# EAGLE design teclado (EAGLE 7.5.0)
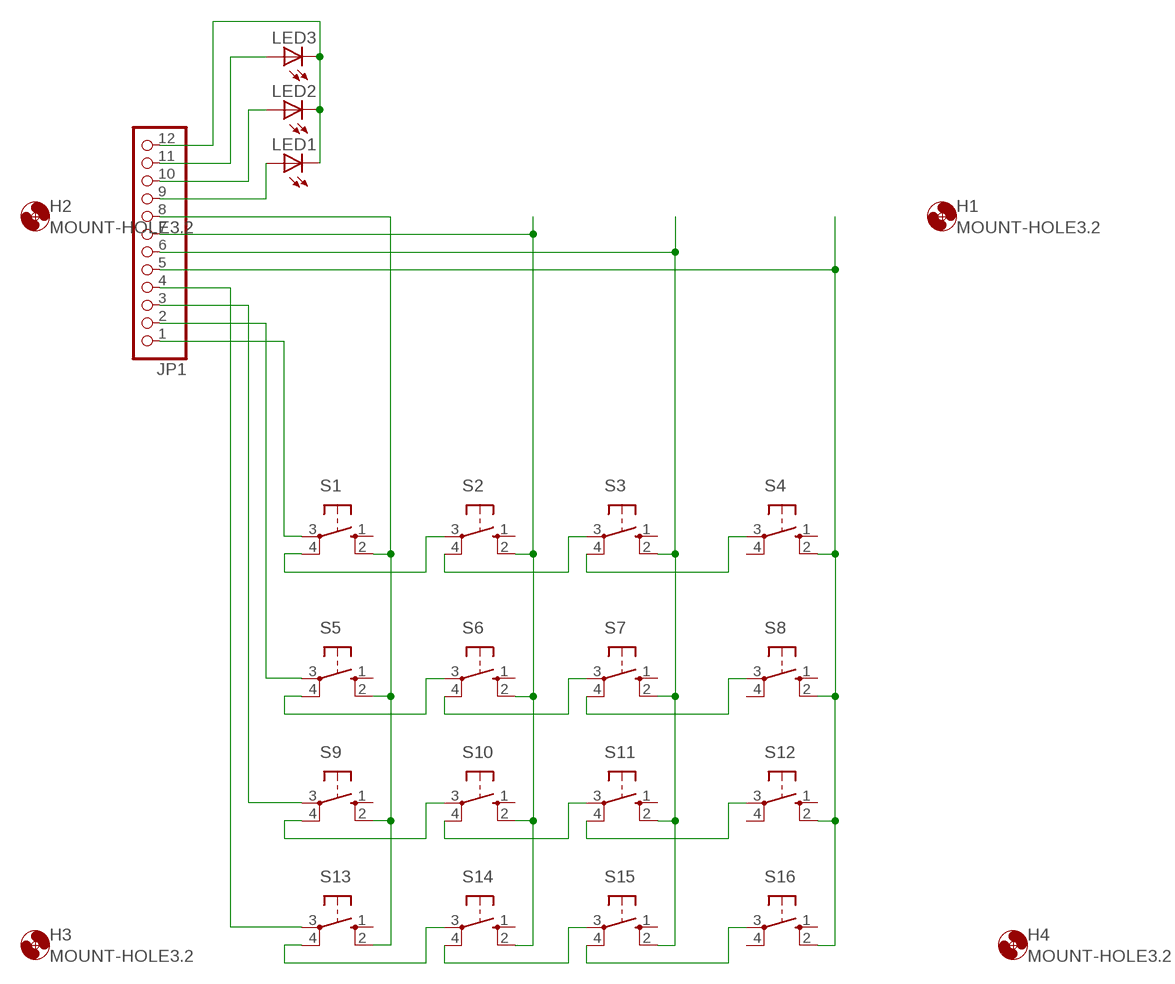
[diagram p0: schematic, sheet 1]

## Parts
H1  MOUNT-HOLE3.2  [3,2]
H2  MOUNT-HOLE3.2  [3,2]
H3  MOUNT-HOLE3.2  [3,2]
H4  MOUNT-HOLE3.2  [3,2]
JP1  PINHD-1X12  [1X12]
LED1  LED5MM  [LED5MM]
LED2  LED5MM  [LED5MM]
LED3  LED5MM  [LED5MM]
S1  10-XX  [B3F-10XX]
S2  10-XX  [B3F-10XX]
S3  10-XX  [B3F-10XX]
S4  10-XX  [B3F-10XX]
S5  10-XX  [B3F-10XX]
S6  10-XX  [B3F-10XX]
S7  10-XX  [B3F-10XX]
S8  10-XX  [B3F-10XX]
S9  10-XX  [B3F-10XX]
S10  10-XX  [B3F-10XX]
S11  10-XX  [B3F-10XX]
S12  10-XX  [B3F-10XX]
S13  10-XX  [B3F-10XX]
S14  10-XX  [B3F-10XX]
S15  10-XX  [B3F-10XX]
S16  10-XX  [B3F-10XX]

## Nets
N$1: JP1.1 S1.3(P)
N$2: JP1.8 S1.2(S1) S5.2(S1) S9.2(S1) S13.2(S1)
N$3: JP1.7 S2.2(S1) S6.2(S1) S10.2(S1) S14.2(S1)
N$4: JP1.6 S3.2(S1) S7.2(S1) S11.2(S1) S15.2(S1)
N$5: JP1.5 S4.2(S1) S8.2(S1) S12.2(S1) S16.2(S1)
N$6: S1.4(P1) S2.3(P)
N$7: S5.4(P1) S6.3(P)
N$8: S9.4(P1) S10.3(P)
N$9: S13.4(P1) S14.3(P)
N$10: S2.4(P1) S3.3(P)
N$11: S6.4(P1) S7.3(P)
N$12: S10.4(P1) S11.3(P)
N$13: S14.4(P1) S15.3(P)
N$14: S3.4(P1) S4.3(P)
N$15: S7.4(P1) S8.3(P)
N$16: S11.4(P1) S12.3(P)
N$17: S15.4(P1) S16.3(P)
N$18: JP1.2 S5.3(P)
N$19: JP1.3 S9.3(P)
N$20: JP1.4 S13.3(P)
N$21: JP1.9 LED1.A
N$22: JP1.10 LED2.A
N$23: JP1.11 LED3.A
N$24: JP1.12 LED1.K(C) LED2.K(C) LED3.K(C)
Unconnected: S1.1(S) S2.1(S) S3.1(S) S4.1(S) S4.4(P1) S5.1(S) S6.1(S) S7.1(S) S8.1(S) S8.4(P1) S9.1(S) S10.1(S) S11.1(S) S12.1(S) S12.4(P1) S13.1(S) S14.1(S) S15.1(S) S16.1(S) S16.4(P1)

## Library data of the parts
H1-H4 = holes:MOUNT-HOLE: MOUNTING HOLE with drill center marker
JP1 = pinhead:PINHD-1X12: PIN HEADER
LED1-LED3 = led:LED: LED
S1-S16 = switch-omron:10-XX: OMRON SWITCH; MPN: B3F-1000; OC_FARNELL: 176432; OC_NEWARK: 36M3542

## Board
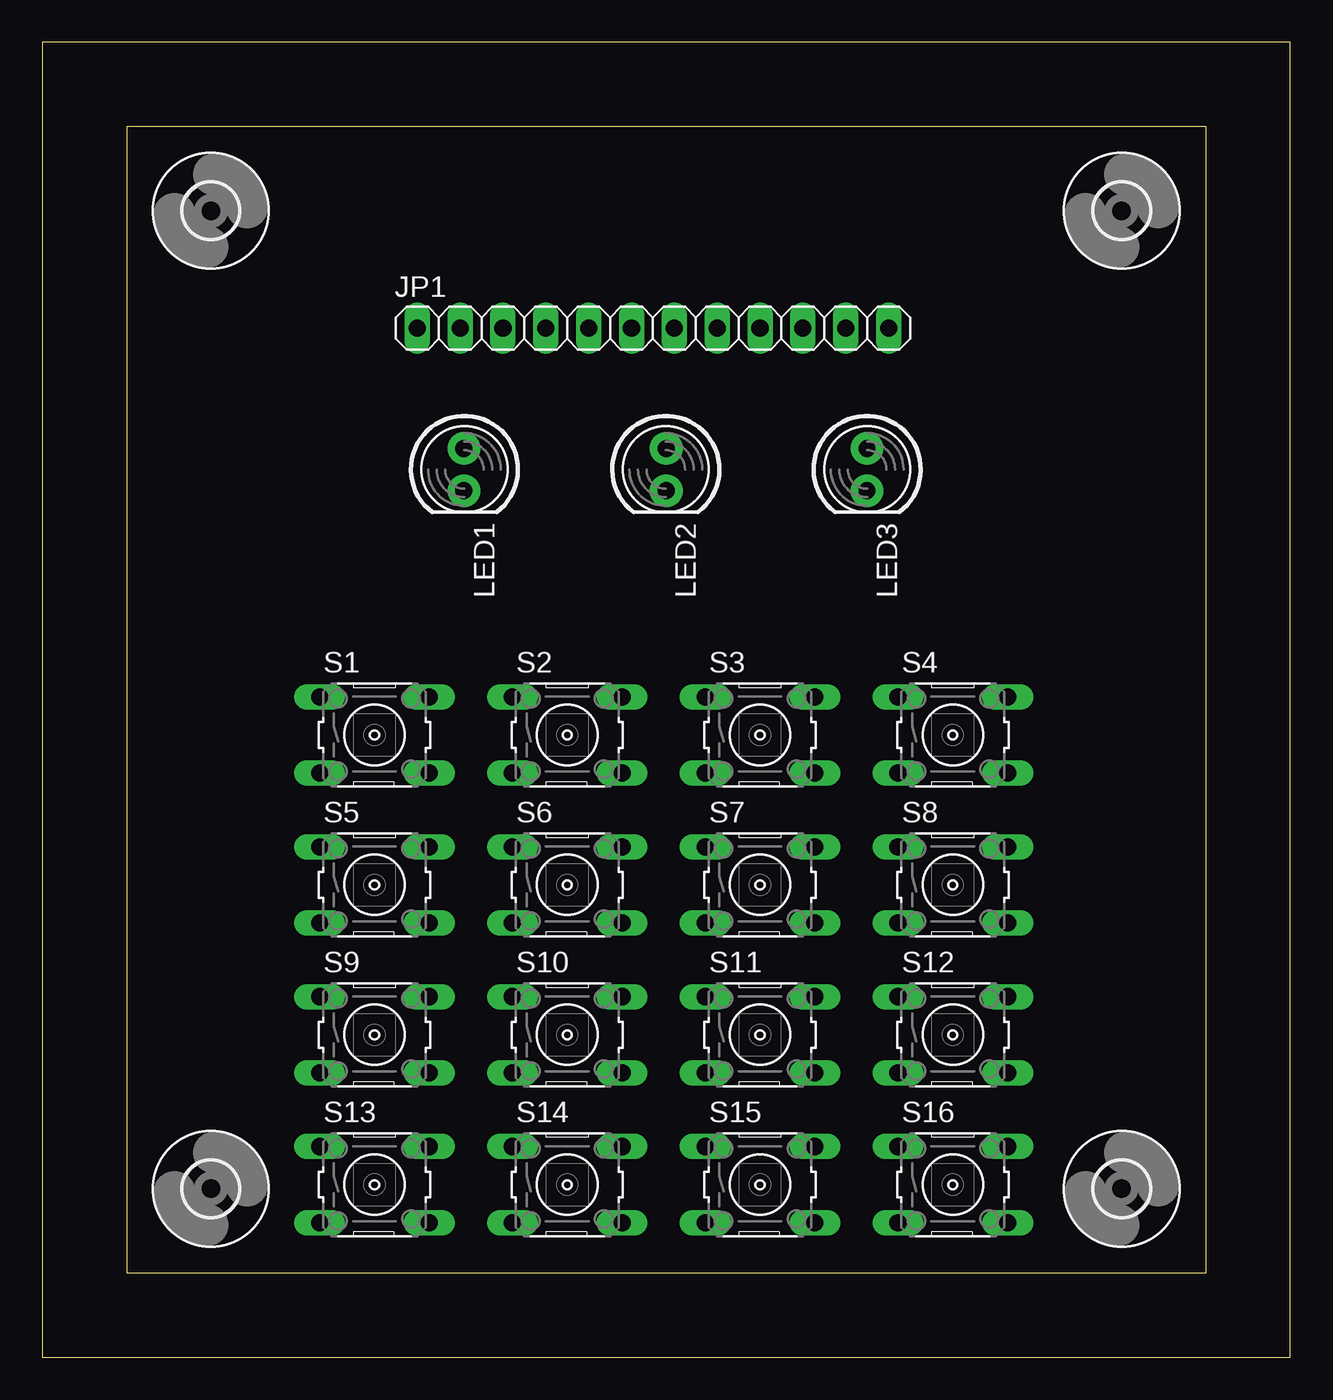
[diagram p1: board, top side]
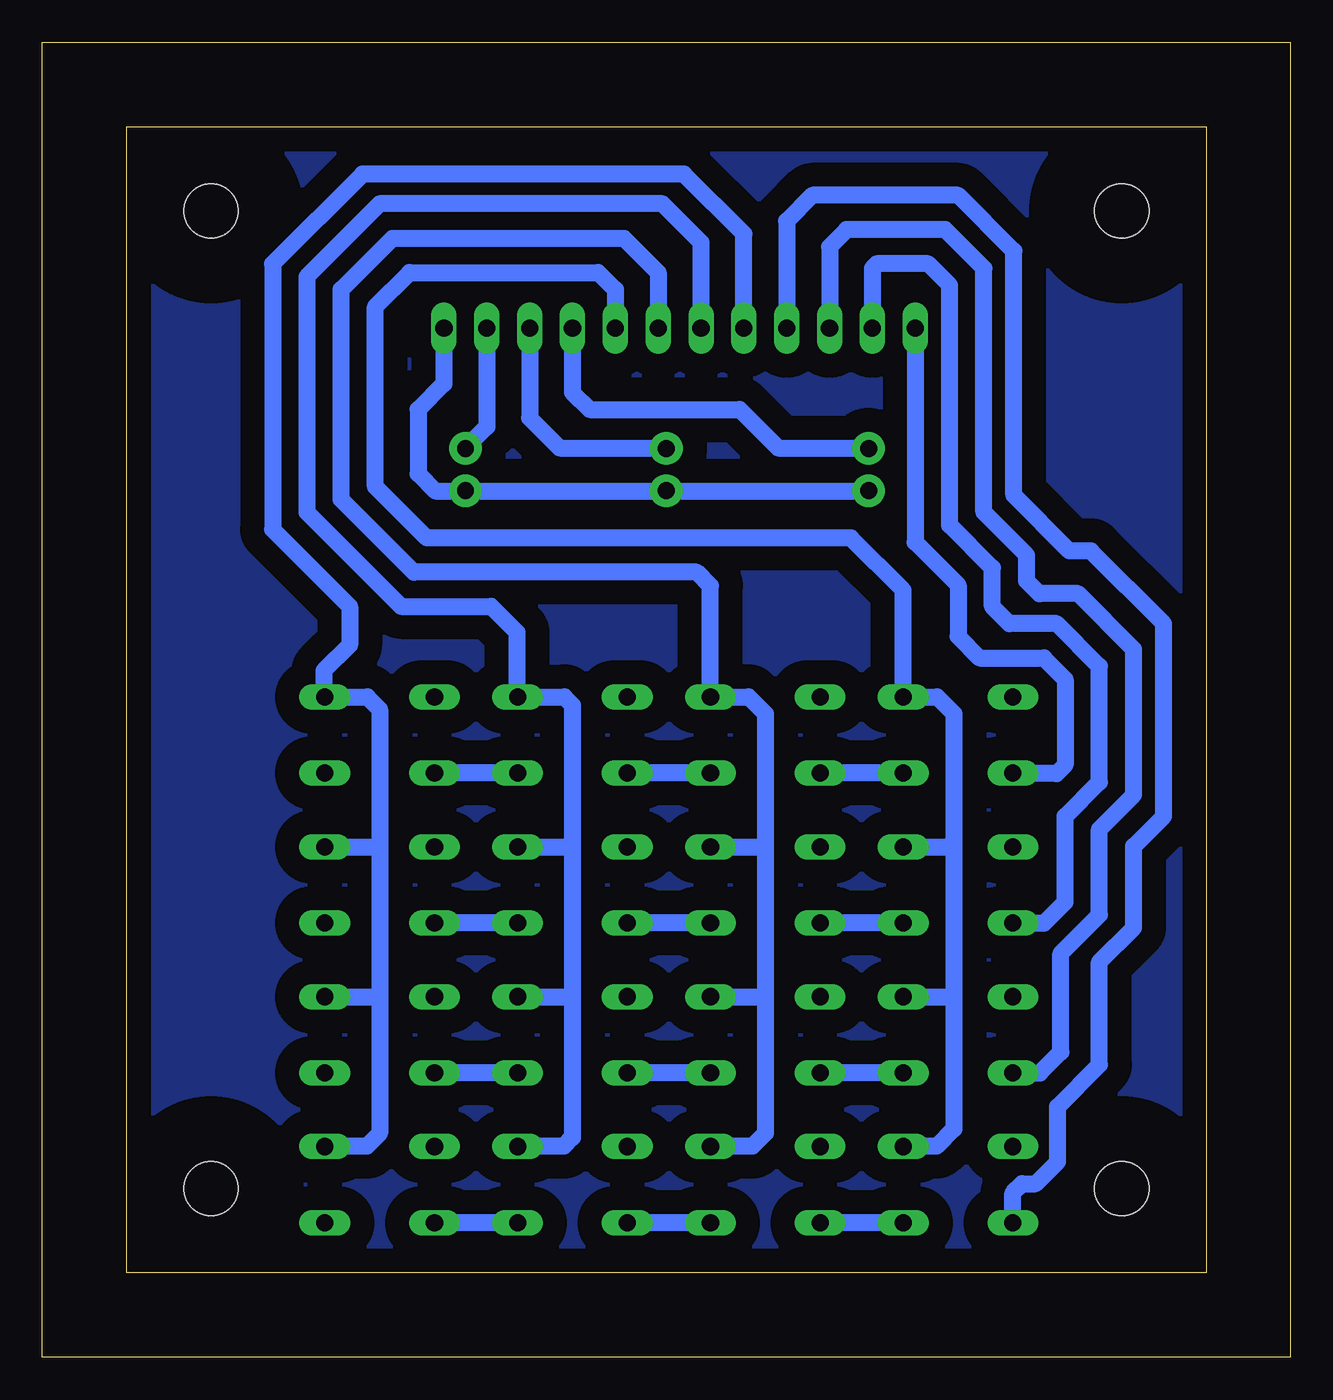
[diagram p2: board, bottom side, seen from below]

Size 74 x 78 mm. Coordinates in mm from the lower left corner, seen from the top.
Outline: 5,5 69,5 69,73 5,73 5,5
Outline: 0,0 74,0 74,78 0,78 0,0
Copper layers (1*16): Top 0.035mm / dielectric 1.5mm / Bottom 0.035mm
Design rules "default": minimum track width 10mil, minimum drill 24mil, track to track 8mil, track to pad 8mil, pad to pad 8mil, via to via 8mil, smd to smd 8mil, copper to edge 40mil, drill to drill 8mil, minimum pad ring 10mil, minimum via ring 8mil, stop-mask expansion 4mil, vias tented up to drill 0mil, thermal gap 10mil

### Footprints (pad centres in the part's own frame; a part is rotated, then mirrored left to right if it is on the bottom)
3,2 = hole 3.2: 0,0
1X12 = drill 1.016 long: 1 -13.97,0; 2 -11.43,0; 3 -8.89,0; 4 -6.35,0; 5 -3.81,0; 6 -1.27,0; 7 1.27,0; 8 3.81,0; 9 6.35,0; 10 8.89,0; 11 11.43,0; 12 13.97,0
LED5MM = drill 0.813 octagon: A -1.27,0; K 1.27,0
B3F-10XX = drill 1.016 long: 1 -3.251,2.261; 2 3.251,2.261; 3 -3.251,-2.261; 4 3.251,-2.261

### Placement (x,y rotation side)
H1  10,68 0 top
H2  64,68 0 top
H3  64,10 0 top
H4  10,10 0 top
JP1  36.21,61.04 0 top
LED1  25.03,52.66 270 top
LED2  36.97,52.66 270 top
LED3  48.91,52.66 270 top
S1  19.7,36.91 0 top
S2  31.13,36.91 0 top
S3  42.56,36.91 0 top
S4  53.99,36.91 0 top
S5  19.7,28.02 0 top
S6  31.13,28.02 0 top
S7  42.56,28.02 0 top
S8  53.99,28.02 0 top
S9  19.7,19.13 0 top
S10  31.13,19.13 0 top
S11  42.56,19.13 0 top
S12  53.99,19.13 0 top
S13  19.7,10.24 0 top
S14  31.13,10.24 0 top
S15  42.56,10.24 0 top
S16  53.99,10.24 0 top

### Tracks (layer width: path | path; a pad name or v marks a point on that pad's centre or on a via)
N$1
  Bottom 1.016: JP1.1 22.24,48.34 19.7,45.8 19.7,42.75 18.43,41.48 14.62,41.48 13.35,40.21 13.35,35.13 13.86,34.62 16.42,34.62 S1.3
N$2
  Bottom 1.016: 19.95,30.56 19.95,38.18 20.95,39.17 S1.2 22.95,45.49 26.05,48.59 51.2,48.59 54.24,51.64 54.24,62.31 52.21,64.34 41.04,64.34 40.02,63.33 JP1.8 | 19.95,30.56 19.95,21.42 | 19.95,21.42 19.95,13.54 20.97,12.53 22.93,12.53 S13.2 | S9.2 19.98,21.39 19.95,21.42 | S5.2 20.23,30.28 19.95,30.56
N$3
  Bottom 1.016: 31.13,30.05 31.13,38.18 32.12,39.17 S2.2 34.38,45.75 35.19,46.56 51.96,46.56 56.28,50.88 56.28,63.33 53.23,66.37 39.51,66.37 37.48,64.34 JP1.7 | 31.13,30.05 31.13,21.42 | 31.13,21.42 31.13,13.29 31.89,12.53 34.36,12.53 S14.2 | S10.2 31.16,21.39 31.13,21.42 | S6.2 31.36,30.28 31.13,30.05
N$4
  Bottom 1.016: 42.56,30.56 42.56,38.69 43.04,39.17 S3.2 45.86,39.22 45.86,43.01 47.39,44.53 52.72,44.53 58.31,50.12 58.31,64.09 53.99,68.41 37.23,68.41 34.94,66.12 JP1.6 | 42.56,30.56 42.56,21.42 | 42.56,21.42 42.56,13.03 43.07,12.53 45.79,12.53 S15.2 | S11.2 42.59,21.39 42.56,21.42 | S7.2 42.84,30.28 42.56,30.56
N$5
  Bottom 1.016: 53.99,30.31 53.99,38.43 54.73,39.17 S4.2 57.29,39.22 57.29,40.72 55.77,42.24 55.77,44.53 60.34,49.1 60.34,64.85 55.01,70.18 35.96,70.18 32.4,66.63 JP1.5 | 53.99,30.31 53.99,21.16 | 53.99,21.16 53.99,13.29 54.75,12.53 57.22,12.53 S16.2 | S12.2 54.22,21.39 53.99,21.16 | S8.2 54.02,30.28 53.99,30.31
N$6
  Bottom 1.016: S1.4 S2.3
N$7
  Bottom 1.016: S5.4 S6.3
N$8
  Bottom 1.016: S9.4 S10.3
N$9
  Bottom 1.016: S13.4 S14.3
N$10
  Bottom 1.016: S2.4 S3.3
N$11
  Bottom 1.016: S6.4 S7.3
N$12
  Bottom 1.016: S10.4 S11.3
N$13
  Bottom 1.016: S14.4 S15.3
N$14
  Bottom 1.016: S3.4 S4.3
N$15
  Bottom 1.016: S7.4 S8.3
N$16
  Bottom 1.016: S11.4 S12.3
N$17
  Bottom 1.016: S15.4 S16.3
N$18
  Bottom 1.016: S5.3 14.6,25.76 13.35,27 13.35,32.08 11.32,34.12 11.32,40.97 13.86,43.51 16.65,43.51 17.67,44.53 17.67,46.82 20.21,49.36 20.21,63.58 21.48,64.85 24.53,64.85 24.78,64.6 JP1.2
N$19
  Bottom 1.016: S9.3 14.85,16.87 13.6,18.11 13.6,23.96 11.32,26.24 11.32,31.32 9.29,33.35 9.29,41.99 12.59,45.29 14.87,45.29 15.64,46.05 15.64,47.58 18.18,50.12 18.18,64.6 20.46,66.88 26.3,66.88 27.32,65.87 JP1.3
N$20
  Bottom 1.016: JP1.4 29.86,67.39 28.34,68.91 19.7,68.91 16.4,65.61 16.4,51.13 13.1,47.83 11.83,47.83 7.51,43.51 7.51,32.08 9.29,30.31 9.29,25.48 11.32,23.45 11.32,17.35 13.8,14.87 13.8,11.6 15.1,10.3 15.9,10.3 16.45,9.75 S13.3
N$21
  Bottom 1.016: JP1.9 42.56,57.23 41.54,56.21 32.65,56.21 30.37,53.93 LED1.A
N$22
  Bottom 1.016: JP1.10 45.1,55.71 43.32,53.93 LED2.A
N$23
  Bottom 1.016: JP1.11 47.64,55.2 LED3.A
N$24
  Bottom 1.016: JP1.12 50.18,57.74 51.7,56.21 51.7,52.4 50.69,51.39 LED3.K LED2.K LED1.K
N$26
  pour Bottom (isolate 1.422): 6,72 68,72 68,6 6,6
N$27  (via drill 1 pad 1.93)
  other vias: 25,51.4
N$28  (via drill 1 pad 1.93)
  other vias: 25,53.9
N$29  (via drill 1 pad 1.93)
  other vias: 37,51.4
N$30  (via drill 1 pad 1.93)
  other vias: 37,53.9
N$31  (via drill 1 pad 1.93)
  other vias: 48.9,51.4
N$32  (via drill 1 pad 1.93)
  other vias: 48.9,53.9

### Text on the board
tTest: F1 | F2 | F3 | F4 | C4 | C3 | C2 | C1 | POWER | PROC | READY | GND | POWER PROC READY | 1 2 3 A | 4 5 6 B | 7 8 9 C | * 0 # D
